{attribute 'pack_mode' := '0'}
TYPE TPTP_DIAG :
STRUCT
   PTPVersion				: E_PTP_VERSION;
   PTPState					: E_PTP_PORT_STATE;
   ClockIdentity			: ARRAY [0..7] OF USINT;
   ParentPortIdentity		: ARRAY [0..9] OF USINT;
   GrandmasterIdentity		: ARRAY [0..7] OF USINT;
   OffsetFromMaster			: DINT;
   MeanPathDelay			: UDINT;
   StepsRemoved				: UINT;
   SyncEventSequenceNumber	: UINT;
   Timescale				: UINT;
   CurrentUtcOffset			: INT;
   CurrentUtcOffsetIsValid	: UINT; 
   Leap61					: UINT;
   Leap59					: UINT;
   Epoch_Number				: UINT;
END_STRUCT
END_TYPE
